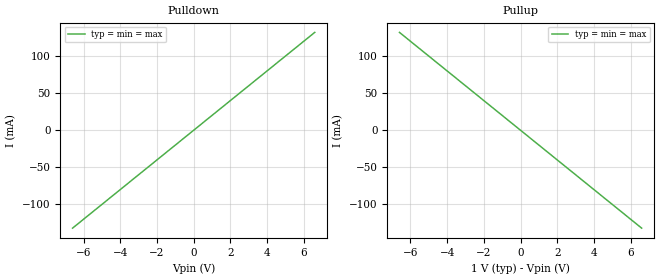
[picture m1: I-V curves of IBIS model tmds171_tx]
[IBIS Ver]   5.0
[File Name]   tmds171.ibs
[File Rev]   1.0
[Component]   tmds171_tx
[Manufacturer] My Company
[Package]
R_pkg  0.0   NA   NA
L_pkg  0.0   NA   NA
C_pkg  0.0   NA   NA
[Pin]   signal_name   model_name   R_pin L_pin  C_pin
1p   tmds171_tx_p   tmds171_tx
1n   tmds171_tx_n   tmds171_tx
2p   tmds171_rx_2p   tmds171_rx
2n   tmds171_rx_2n   tmds171_rx
[Diff_Pin] inv_pin vdiff tdelay_typ tdelay_min tdelay_max
1p   1n   NA   NA   NA   NA
2p   2n   NA   NA   NA   NA
[Model] tmds171_rx
Model_type Input
C_comp 0p 0p 0p
Vinh = 0.25
Vinl = -0.25
[Temperature_Range] 25 125 0
[Voltage Range] 1.0 1.0 1.0
[Algorithmic Model]
Executable Windows_cl17.00.50727.1_64 tmds171_rx_x64.dll tmds171_rx.ami
Executable Windows_cl17.00.50727.1_32 tmds171_rx.dll tmds171_rx.ami
[End Algorithmic Model]
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| Models and submodels in the file (2): tmds171_tx (Output), tmds171_rx (Input)
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[Model] tmds171_tx
Model_type Output
C_comp 0p 0p 0p
Cref = 0
Vref = 0.5
Rref = 50
Vmeas = 0.5
[Temperature_Range] 25 125 0
[Voltage Range] 1.0 1.0 1.0
[Algorithmic Model]
Executable Windows_cl17.00.50727.1_64 tmds171_tx_x64.dll tmds171_tx.ami
Executable Windows_cl17.00.50727.1_32 tmds171_tx.dll tmds171_tx.ami
[End Algorithmic Model]
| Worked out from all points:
|   slope of the pulldown table from 0 to 0.15 V, typ, clamps not added: 50 ohm
|   slope of the pullup table from 0 to 0.15 V, typ, clamps not added: 50 ohm
[Pulldown]
-6.6V     -132mA     -132mA     -132mA
0V        0A         0A         0A
6.6V      132mA      132mA      132mA
[Pullup]
-6.6V     132mA      132mA      132mA
0V        0A         0A         0A
6.6V      -132mA     -132mA     -132mA
[GND Clamp]
-6.6V     0A         0A         0A
0V        0A         0A         0A
6.6V      0A         0A         0A
[Power Clamp]
-6.6V     0A         0A         0A
0V        0A         0A         0A
6.6V      0A         0A         0A
[Ramp]
dV/dt_r 0.3/1.5p 0.3/1.5p 0.3/1.5p
dV/dt_f 0.3/1.5p 0.3/1.5p 0.3/1.5p
